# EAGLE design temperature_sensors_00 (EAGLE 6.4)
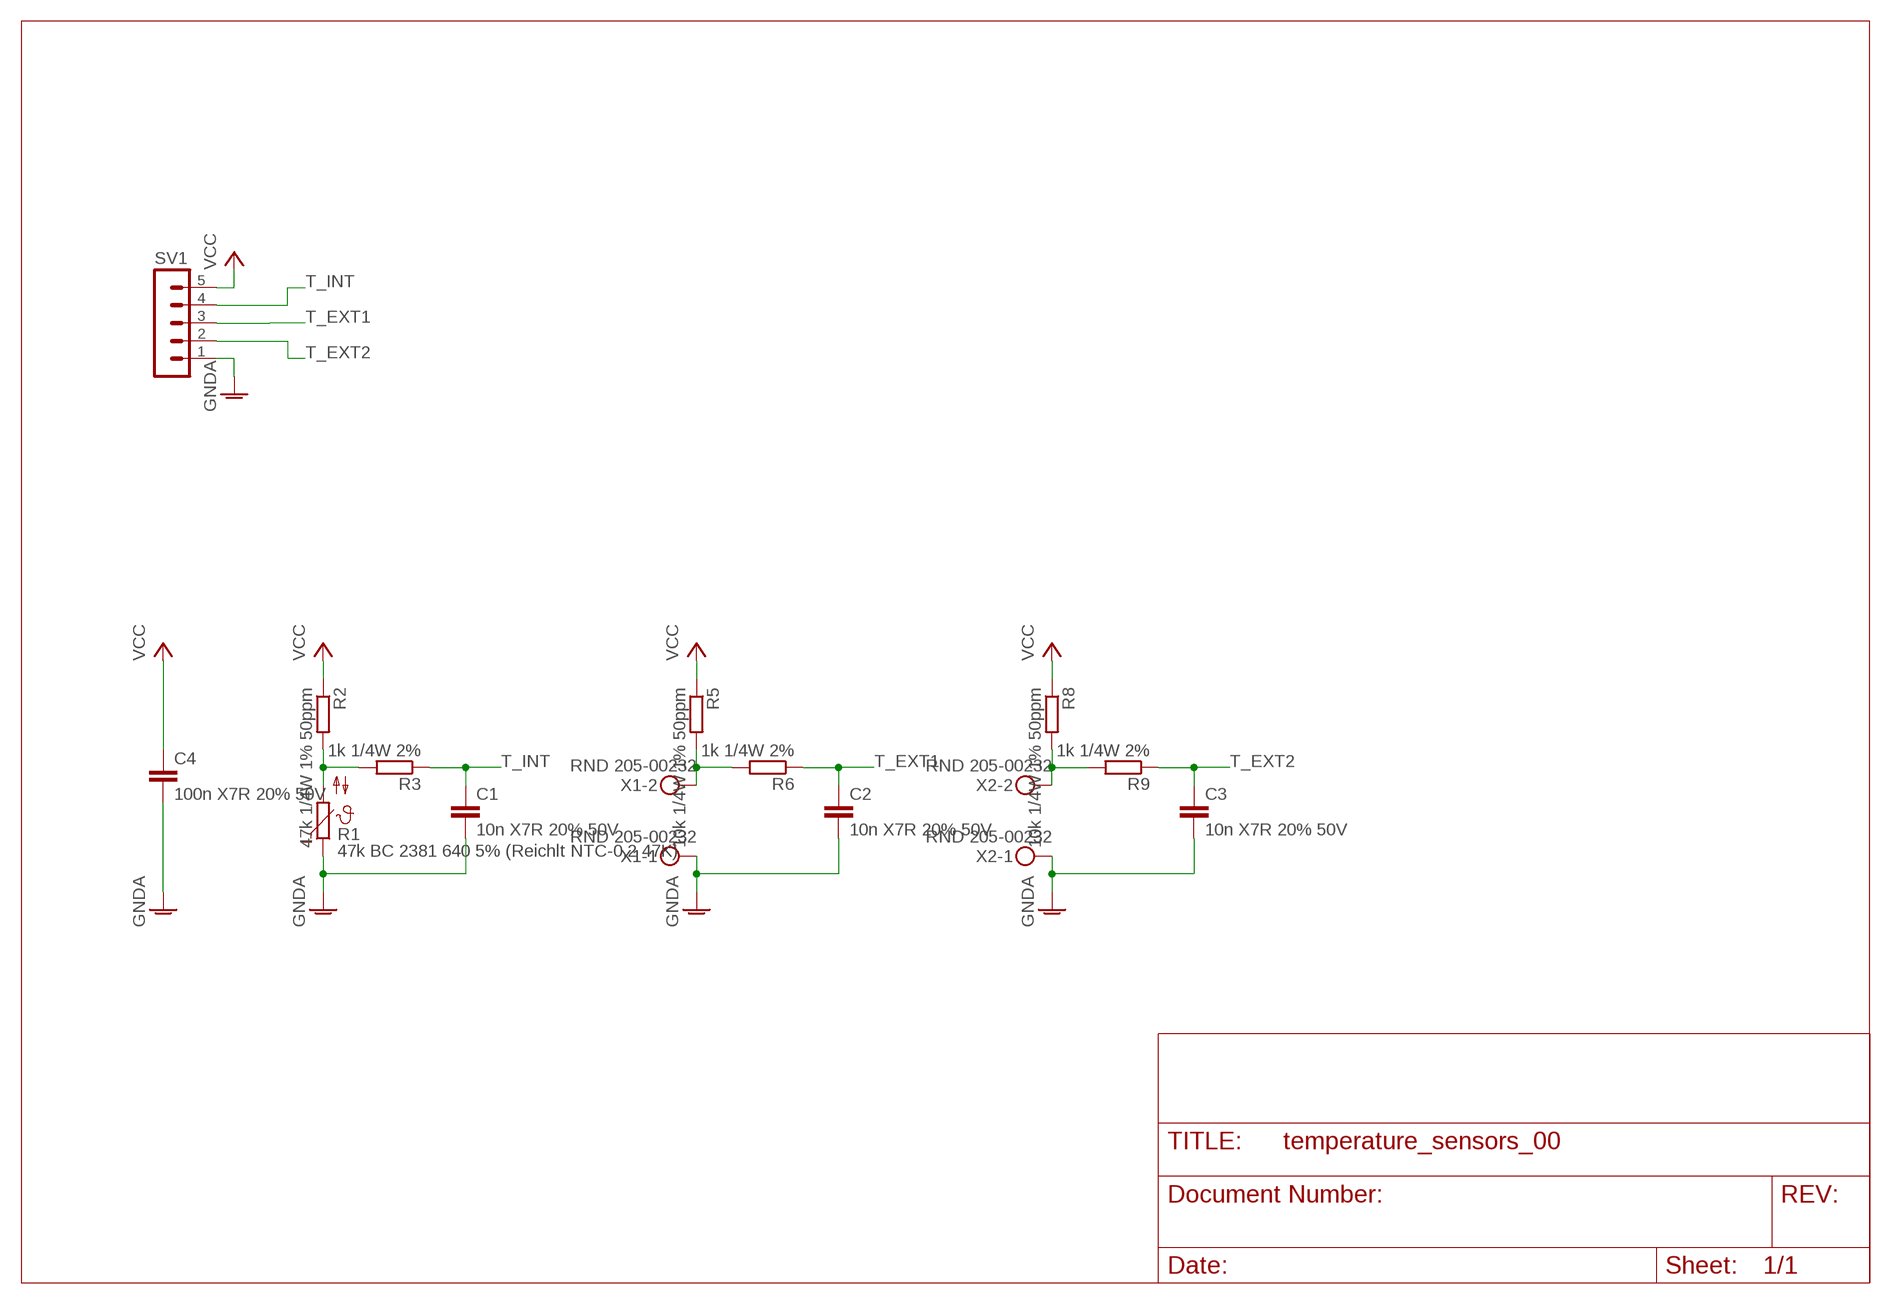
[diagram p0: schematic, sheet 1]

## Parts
C1  10n X7R 20% 50V  C-EU025-025X050  [C025-025X050]
C2  10n X7R 20% 50V  C-EU025-025X050  [C025-025X050]
C3  10n X7R 20% 50V  C-EU025-025X050  [C025-025X050]
C4  100n X7R 20% 50V  C-EU025-025X050  [C025-025X050]
R1  47k BC 2381 640 5% (Reichlt NTC-0,2 47K)  B57164  [B57164]
R2  47k 1/4W 1% 50ppm  R-EU_0207/10  [0207/10]
R3  1k 1/4W 2%  R-EU_0207/10  [0207/10]
R5  10k 1/4W 1% 50ppm  R-EU_0207/10  [0207/10]
R6  1k 1/4W 2%  R-EU_0207/10  [0207/10]
R8  10k 1/4W 1% 50ppm  R-EU_0207/10  [0207/10]
R9  1k 1/4W 2%  R-EU_0207/10  [0207/10]
SV1  MA05-1  [MA05-1]
X1  RND 205-00232  MKDSN1,5/2-5,08  [MKDSN1,5/2-5,08]
X2  RND 205-00232  MKDSN1,5/2-5,08  [MKDSN1,5/2-5,08]

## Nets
GNDA: C1.2 C2.2 C3.2 C4.2 R1.1 SV1.1 X1.1 X2.1
N$1: R1.2 R2.2 R3.2
N$5: R8.2 R9.2 X2.2
N$7: R5.2 R6.2 X1.2
T_EXT1: C2.1 R6.1 SV1.3
T_EXT2: C3.1 R9.1 SV1.2
T_INT: C1.1 R3.1 SV1.4
VCC: C4.1 R2.1 R5.1 R8.1 SV1.5

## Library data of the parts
C1-C4 = rcl:C-EU: CAPACITOR, European symbol
R1 = ptc-ntc:B57164: SIEMENS NTC; MPN: B57164K474K52; OC_FARNELL: 9753451; OC_NEWARK: 29M3118
R2 R3 R5 R6 R8 R9 = rcl:R-EU_: RESISTOR, European symbol; OC_REICHELT: 1/4W; PART_VALUE: 1/4W 5%
SV1 = con-lstb:MA05-1: PIN HEADER; OC_FARNELL: unknown; OC_NEWARK: unknown
X1 X2 = con-phoenix-508:MKDSN1,5/2-5,08: MKDSN 1,5/ 2-5,08 Printklemme; MPN: MKDSN 1,5/2-5.08; OC_FARNELL: 1792903; OC_NEWARK: 30M2397

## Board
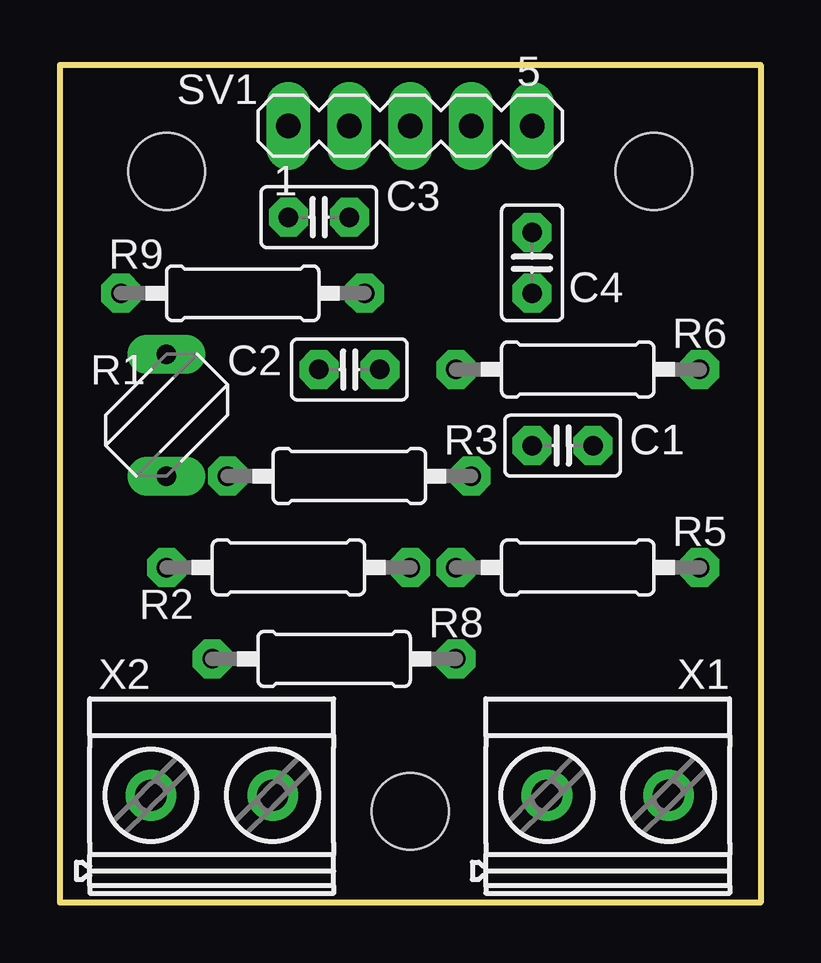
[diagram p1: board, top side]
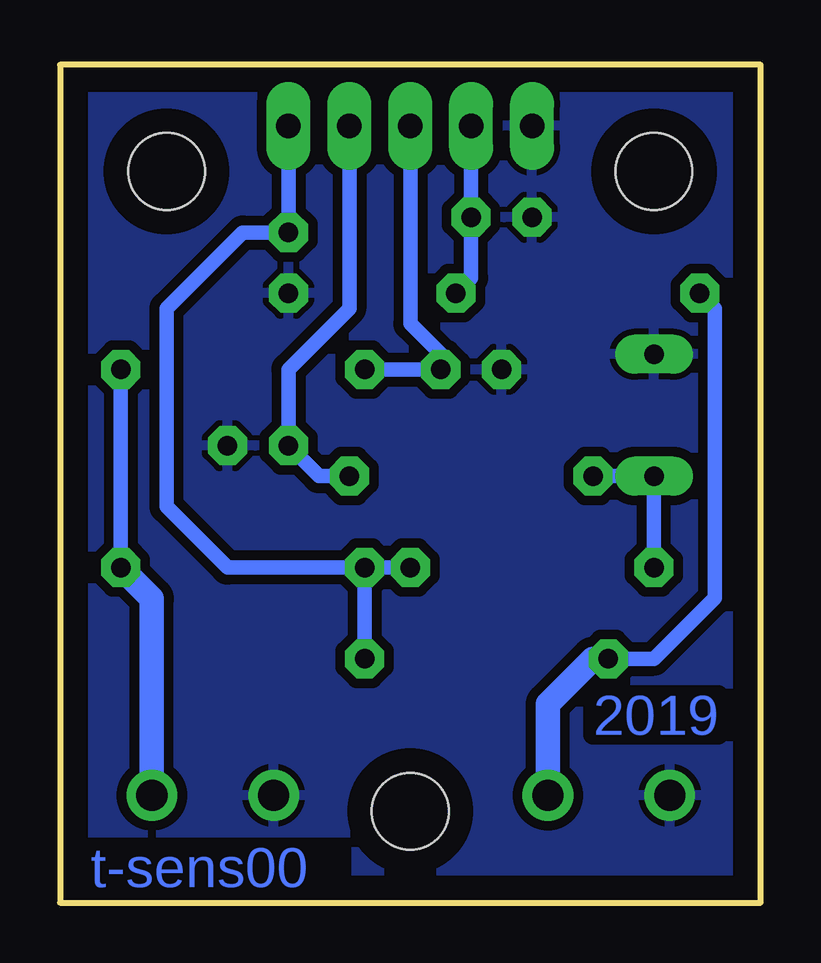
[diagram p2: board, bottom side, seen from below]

Size 29.21 x 34.92 mm. Coordinates in mm from the lower left corner, seen from the top.
Outline: 0,0 0,34.92 29.21,34.92 29.21,0 0,0
Copper layers (1*16): Top 0.035mm / dielectric 1.5mm / Bottom 0.035mm
Design rules "later_toner_transfer": minimum track width 10mil, minimum drill 24mil, track to track 16mil, track to pad 16mil, pad to pad 16mil, via to via 16mil, smd to smd 16mil, copper to edge 40mil, drill to drill 16mil, minimum pad ring 16mil, minimum via ring 16mil, stop-mask expansion 4mil, vias tented up to drill 0mil, thermal gap 10mil
Holes 3.2 mm at 4.45,30.48 24.77,30.48 14.61,3.81

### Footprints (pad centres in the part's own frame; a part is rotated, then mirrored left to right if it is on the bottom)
C025-025X050 = drill 0.813 octagon: 1 -1.27,0; 2 1.27,0
B57164 = drill 0.813 long: 1 -2.54,0; 2 2.54,0
0207/10 = drill 0.813 octagon: 1 -5.08,0; 2 5.08,0
MA05-1 = drill 1.016 long: 1 -5.08,0; 2 -2.54,0; 3 0,0; 4 2.54,0; 5 5.08,0
MKDSN1,5/2-5,08 = drill 1.3 pad 2: 1 -2.561,0.025; 2 2.519,0.025

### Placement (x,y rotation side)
C1  20.95,19.05 0 top
C2  12.06,22.23 180 top
C3  10.79,28.57 180 top
C4  19.68,26.67 270 top
R1  4.45,20.32 270 top
R2  9.53,13.97 180 top
R3  12.06,17.78 180 top
R5  21.59,13.97 0 top
R6  21.59,22.23 0 top
R8  11.43,10.16 180 top
R9  7.62,25.4 180 top
SV1  14.61,32.38 0 top
X1  22.86,4.45 0 top
X2  6.35,4.45 0 top

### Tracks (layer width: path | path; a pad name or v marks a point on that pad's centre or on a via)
GNDA
  pour Bottom: 0.64,0.64 0.64,34.29 28.57,34.29 28.57,0.64
N$1
  Bottom 0.61: R2.2 R1.2 R3.2
N$2  (via drill 1)
  other vias: 4.45,30.48
N$3  (via drill 1)
  other vias: 24.77,30.48
N$4  (via drill 1)
  other vias: 14.61,3.81
N$5
  Bottom 0.61: R9.2 1.91,24.77 1.91,12.7 4.45,10.16 R8.2
  Bottom 1.016: X2.2 8.87,8.28 6.99,10.16 R8.2
N$7
  Bottom 0.61: R6.2 R5.2
  Bottom 1.016: X1.2 25.38,12.68 R5.2
T_EXT1
  Bottom 0.61: SV1.3 14.61,24.13 13.34,22.86 C2.1 R6.1
T_EXT2
  Bottom 0.61: R9.1 12.06,26.04 C3.1 SV1.2
T_INT
  Bottom 0.61: SV1.4 17.14,24.77 19.68,22.23 C1.1 18.41,17.78 R3.1
VCC
  Bottom 0.61: R5.1 R8.1 | SV1.5 C4.1 21.59,27.94 24.77,24.77 24.77,16.51 22.23,13.97 R5.1 | R2.1 R5.1

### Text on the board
Bottom: 2019 | t-sens00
